FUNCTION FC_REAL_DEAL : REAL
VAR_INPUT
	
	In_lreal: LREAL;(*输入值*)
	In_usint: INT; (*输入保留小数位数*)
	
END_VAR
VAR
END_VAR

In_usint:=LIMIT(0,In_usint,5); (*本程序限制最多精确到小数点后面第5位,用户可根据自己的需求修改*) 

FC_REAL_DEAL:=LREAL_TO_DINT(In_lreal*EXPT(10,In_usint) )/EXPT(10,In_usint);

END_FUNCTION
